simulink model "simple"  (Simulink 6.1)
settings: Solver=ode45  StartTime=0.0  StopTime=25.0  RelTol=1e-3
undefined symbols (not defined in the file or in its folder): Bit, Location, Lower, simple_netlist, Width
libraries: xbsIndex_r3 x16, adlibrary2 x1

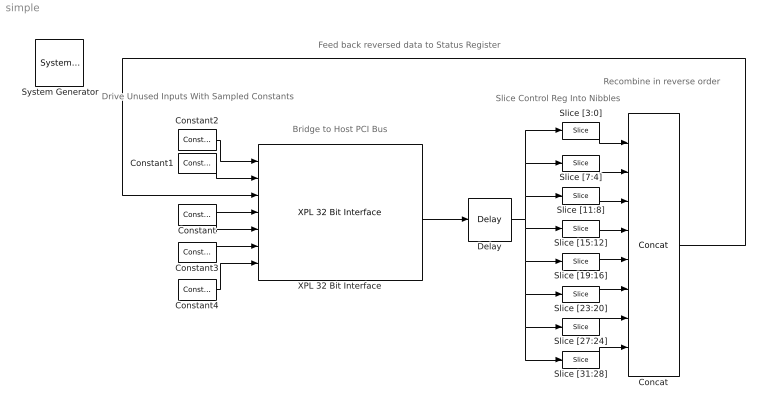
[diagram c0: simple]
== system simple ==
  note: Drive Unused Inputs With Sampled Constants
  note: Bridge to Host PCI Bus
  note: Slice Control Reg Into Nibbles
  note: Recombine in reverse order
  note: Feed back reversed data to Status Register
  " System Generator" : xbsIndex_r3/ System Generator  Tag=genX  xilinxfamily=Virtex2P  part=xc2vp30  speed=-6  package=ff896  synthesis_tool=XST  directory=./simple_netlist  testbench=off  simulink_period=1  sysclk_period=7.5  incr_netlist=off  trim_vbits=Everywhere in SubSystem  dbl_ovrd=According to Block Masks  core_generation=According to Block Masks  run_coregen=off  deprecated_control=off  eval_field=0
  Concat : xbsIndex_r3/Concat  num_inputs=8  explicit_period=off  period=1  dbl_ovrd=off
  Constant : xbsIndex_r3/Constant  const=0  equ=P=C  arith_type=Boolean  n_bits=1  bin_pt=0  opselect=C  inp2=PCIN>>17  opr=+  inp1=P  carry=CIN  iostate=0  explicit_period=on  period=1  dbl_ovrd=off
  Constant1 : xbsIndex_r3/Constant  const=1  equ=P=C  arith_type=Boolean  n_bits=1  bin_pt=0  opselect=C  inp2=PCIN>>17  opr=+  inp1=P  carry=CIN  iostate=0  explicit_period=on  period=1  dbl_ovrd=off
  Constant2 : xbsIndex_r3/Constant  const=0  equ=P=C  arith_type=Unsigned  n_bits=32  bin_pt=0  opselect=C  inp2=PCIN>>17  opr=+  inp1=P  carry=CIN  iostate=0  explicit_period=on  period=1  dbl_ovrd=off
  Constant3 : xbsIndex_r3/Constant  const=0  equ=P=C  arith_type=Unsigned  n_bits=32  bin_pt=0  opselect=C  inp2=PCIN>>17  opr=+  inp1=P  carry=CIN  iostate=0  explicit_period=on  period=1  dbl_ovrd=off
  Constant4 : xbsIndex_r3/Constant  const=0  equ=P=C  arith_type=Unsigned  n_bits=66  bin_pt=0  opselect=C  inp2=PCIN>>17  opr=+  inp1=P  carry=CIN  iostate=0  explicit_period=on  period=1  dbl_ovrd=off
  Delay : xbsIndex_r3/Delay  latency=1  reg_retiming=off  explicit_period=on  period=1  en=off  accept_only_valid=off  init_zero=on  dbl_ovrd=off  show_param=off
  Slice [11:8] : xbsIndex_r3/Slice  mode=Lower Bit Location + Width  nbits=4  bit1=0  base1=MSB of Input  bit0=8  base0=LSB of Input  boolean_output=off  explicit_period=off  period=1  dbl_ovrd=off
  Slice [15:12] : xbsIndex_r3/Slice  mode=Lower Bit Location + Width  nbits=4  bit1=0  base1=MSB of Input  bit0=12  base0=LSB of Input  boolean_output=off  explicit_period=off  period=1  dbl_ovrd=off
  Slice [19:16] : xbsIndex_r3/Slice  mode=Lower Bit Location + Width  nbits=4  bit1=0  base1=MSB of Input  bit0=16  base0=LSB of Input  boolean_output=off  explicit_period=off  period=1  dbl_ovrd=off
  Slice [23:20] : xbsIndex_r3/Slice  mode=Lower Bit Location + Width  nbits=4  bit1=0  base1=MSB of Input  bit0=20  base0=LSB of Input  boolean_output=off  explicit_period=off  period=1  dbl_ovrd=off
  Slice [27:24] : xbsIndex_r3/Slice  mode=Lower Bit Location + Width  nbits=4  bit1=0  base1=MSB of Input  bit0=24  base0=LSB of Input  boolean_output=off  explicit_period=off  period=1  dbl_ovrd=off
  Slice [31:28] : xbsIndex_r3/Slice  mode=Lower Bit Location + Width  nbits=4  bit1=0  base1=MSB of Input  bit0=28  base0=LSB of Input  boolean_output=off  explicit_period=off  period=1  dbl_ovrd=off
  Slice [3:0] : xbsIndex_r3/Slice  mode=Lower Bit Location + Width  nbits=4  bit1=0  base1=MSB of Input  bit0=0  base0=LSB of Input  boolean_output=off  explicit_period=off  period=1  dbl_ovrd=off
  Slice [7:4] : xbsIndex_r3/Slice  mode=Lower Bit Location + Width  nbits=4  bit1=0  base1=MSB of Input  bit0=4  base0=LSB of Input  boolean_output=off  explicit_period=off  period=1  dbl_ovrd=off
  XPL 32 Bit Interface : adlibrary2/ADM-XPL/XPL 32 Bit Interface  program='slave_write 0x40000 0x1234abcd;slave_read 0x40040'  clock_ratio=1.5
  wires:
  Constant/1 -> XPL 32 Bit Interface/5, XPL 32 Bit Interface/4
  Constant1/1 -> XPL 32 Bit Interface/2
  Constant2/1 -> XPL 32 Bit Interface/1
  Constant3/1 -> XPL 32 Bit Interface/6
  Constant4/1 -> XPL 32 Bit Interface/7
  XPL 32 Bit Interface/6 -> Delay/1
  Delay/1 -> Slice [31:28]/1, Slice [27:24]/1, Slice [23:20]/1, Slice [19:16]/1, Slice [15:12]/1, Slice [11:8]/1, Slice [3:0]/1, Slice [7:4]/1
  Slice [3:0]/1 -> Concat/1
  Slice [7:4]/1 -> Concat/2
  Slice [11:8]/1 -> Concat/3
  Slice [15:12]/1 -> Concat/4
  Slice [19:16]/1 -> Concat/5
  Slice [23:20]/1 -> Concat/6
  Slice [27:24]/1 -> Concat/7
  Slice [31:28]/1 -> Concat/8
  Concat/1 -> XPL 32 Bit Interface/3
